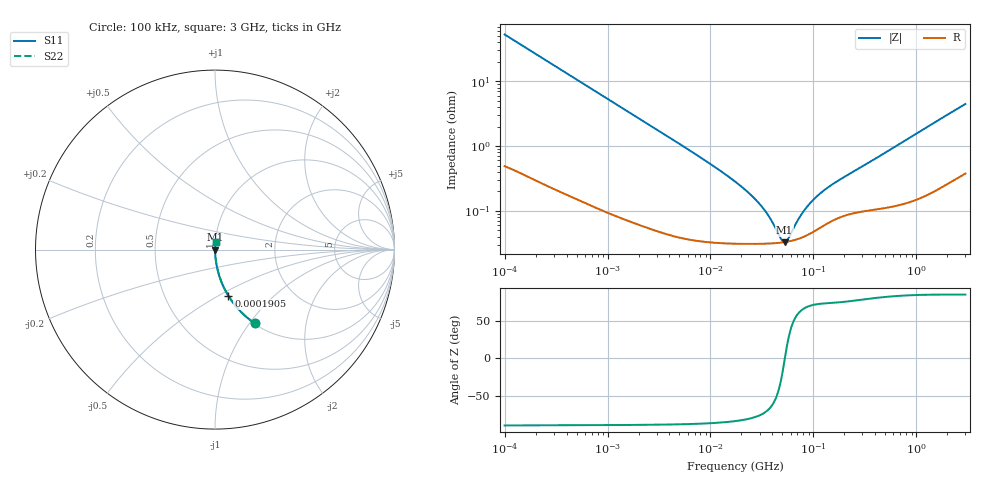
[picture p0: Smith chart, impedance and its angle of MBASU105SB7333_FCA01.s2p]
! MBASU105SB7333_FCA01  S-PARAMETER MODEL  ( Standard Model )
! Model Generated by TAIYO YUDEN Corporation (http://www.ty-top.com)
! Version 2.0
! TAIYO YUDEN Control No. 220822
! Copyright(c) 2021 TAIYO YUDEN CO.,LTD. All Rights Reserved.
! Product Description (link to TY-COMPAS)
! https://ds.yuden.co.jp/TYCOMPAS/or/detail?pn=MBASU105SB7333KFCA01&u=M
! Products Name : Multilayer Ceramic Capacitors
! Characteristics :
!  Capacitance : 0.033 [uF] , Rated Voltage : 50 [V] , TCC : X7R
!  Case Size : 1.0 x 0.5 / 0.039 x 0.02 [mm/inch] , Thickness : 0.5 / 0.02 [mm/inch]
!  (Conditions: Temperature = 25 [degC] , DC Bias Voltage = 0 [V])
! External Node Assignments :
!  1  o---| |---o  2
! GND o---------o GND
! Frequency Range : 100kHz  -  3GHz  [ 401 STEP ]
# MHZ S RI R 50
! Freq[MHz].  S11 Real  S11 Imag  S21 Real  S21 Imag  S12 Real  S12 Imag  S22 Real  S22 Imag
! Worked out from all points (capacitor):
!   401 points, 100 kHz to 3 GHz, reference 50 ohm
!   read as one part in series: C = 30.1 nF near 105.3 kHz
!   lowest |Z| = 32.8 mohm at 52.46 MHz (marker M1)
!   series resonance near 52.83 MHz, so ESL is about 300 pH
!   S11 on the Smith chart (normalised r, x): 100 kHz: 1.01, -1.06; 190.5 kHz: 1.01, -0.56; 3 GHz: 1.01, +0.09
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0.1  0.2204 -0.4099  0.7796 0.4099  0.7796 0.4099  0.2204 -0.4099
0.1398  0.128 -0.329  0.872 0.329  0.872 0.329  0.128 -0.329
0.190467  0.0744 -0.2571  0.9256 0.2571  0.9256 0.2571  0.0744 -0.2571
0.318916  0.029 -0.1618  0.971 0.1618  0.971 0.1618  0.029 -0.1618
0.562235  0.0103 -0.094  0.9897 0.094  0.9897 0.094  0.0103 -0.094
1.18716  0.00288 -0.0451  0.9971 0.0451  0.9971 0.0451  0.00288 -0.0451
3.161081  0.000765 -0.0171  0.9992 0.0171  0.9992 0.0171  0.000765 -0.0171
9.331111  0.00036 -0.00566  0.9996 0.00566  0.9996 0.00566  0.00036 -0.00566
17.7727  0.000317 -0.00273  0.9997 0.00273  0.9997 0.00273  0.000317 -0.00273
24.21403  0.000311 -0.00179  0.9997 0.00179  0.9997 0.00179  0.000311 -0.00179
31.3325  0.00031 -0.00114  0.9997 0.00114  0.9997 0.00114  0.00031 -0.00114
38.50681  0.000313 -0.000669  0.9997 0.000669  0.9997 0.000669  0.000313 -0.000669
48.55934  0.000323 -0.000176  0.9997 0.000176  0.9997 0.000176  0.000323 -0.000176
52.46276  0.000328 -1.45e-05  0.9997 1.45e-05  0.9997 1.45e-05  0.000328 -1.45e-05
56.67997  0.000335 0.000147  0.9997 -0.000147  0.9997 -0.000147  0.000335 0.000147
75.25761  0.00038 0.000754  0.9996 -0.000754  0.9996 -0.000754  0.00038 0.000754
85.60801  0.000416 0.00104  0.9996 -0.00104  0.9996 -0.00104  0.000416 0.00104
97.38194  0.000463 0.00134  0.9995 -0.00134  0.9995 -0.00134  0.000463 0.00134
119.6798  0.000564 0.00184  0.9994 -0.00184  0.9994 -0.00184  0.000564 0.00184
154.8634  0.000713 0.00249  0.9993 -0.00249  0.9993 -0.00249  0.000713 0.00249
547.5153  0.00121 0.00853  0.9988 -0.00853  0.9988 -0.00853  0.00121 0.00853
3000  0.00569 0.044  0.9943 -0.044  0.9943 -0.044  0.00569 0.044
